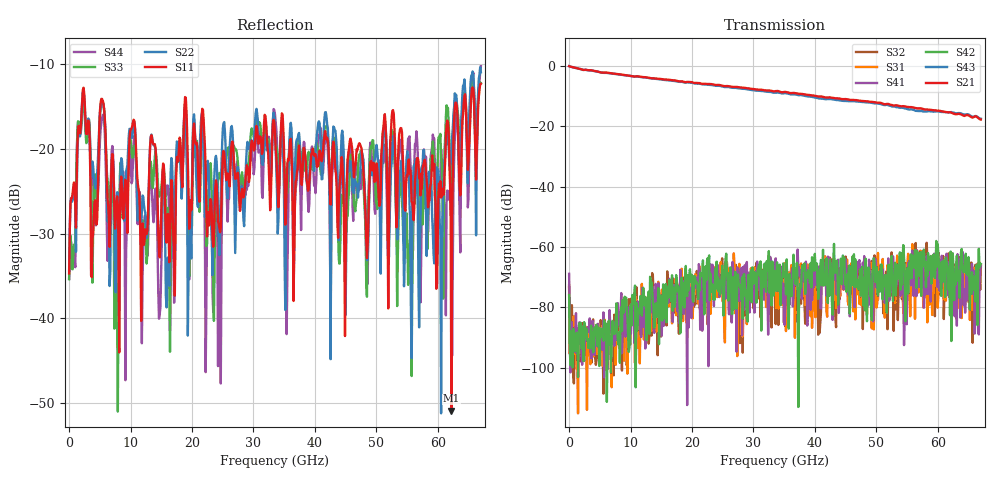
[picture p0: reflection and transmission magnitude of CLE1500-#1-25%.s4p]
!Keysight Technologies,N5247B,US50470101,A.16.20.02
!Date: Thursday, March 13, 2025 10:15:24
!Correction: S11(C  4-Port  )
!S12(C  4-Port  )
!S13(C  4-Port  )
!S14(C  4-Port  )
!S21(C  4-Port  )
!S22(C  4-Port  )
!S23(C  4-Port  )
!S24(C  4-Port  )
!S31(C  4-Port  )
!S32(C  4-Port  )
!S33(C  4-Port  )
!S34(C  4-Port  )
!S41(C  4-Port  )
!S42(C  4-Port  )
!S43(C  4-Port  )
!S44(C  4-Port  )
!S4P File: Measurements: <S11,S12,S13,S14>,
!<S21,S22,S23,S24>,
!<S31,S32,S33,S34>,
!<S41,S42,S43,S44>:
# Hz S  dB  R 50
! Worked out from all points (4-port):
!   601 points, 10 MHz to 67 GHz, reference 50 ohm
!   strongest paths, dB at 10 MHz, 16.76 GHz, 33.51 GHz, 50.25 GHz, 67 GHz:
!     S21: 0.0, -4.7, -8.3, -12.1, -17.7
!     S43: 0.0, -4.9, -8.8, -12.4, -17.5
!     S42: -76.0, -69.4, -68.0, -76.1, -65.6
!     S41: -68.9, -74.0, -71.9, -72.7, -66.2
!     S31: -72.8, -85.3, -66.9, -62.0, -66.1
!     S32: -73.3, -83.8, -70.6, -77.6, -66.8
!   lowest |S11| = -50.9 dB at 62.2 GHz (marker M1), VSWR 1.01, Z = 49.7 + j0.128 ohm
!   |S11| at or under -10 dB: start of sweep to end of sweep
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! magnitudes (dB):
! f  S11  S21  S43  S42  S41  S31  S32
! 10 MHz  -34.7  0.0  0.0  -76.0  -68.9  -72.8  -73.3
! 2.355 GHz  -12.7  -1.2  -1.3  -97.9  -96.8  -93.0  -91.0
! 7.714 GHz  -26.3  -2.6  -2.6  -78.7  -90.8  -82.5  -88.1
! 10.17 GHz  -17.5  -3.3  -3.3  -86.0  -81.7  -81.2  -79.1
! 15.98 GHz  -29.1  -4.4  -4.7  -75.7  -75.5  -74.1  -68.1
! 62.2 GHz  -50.9  -15.4  -15.2  -91.2  -83.6  -67.4  -67.1
! 67 GHz  -12.3  -17.7  -17.5  -65.6  -66.2  -66.1  -66.8
